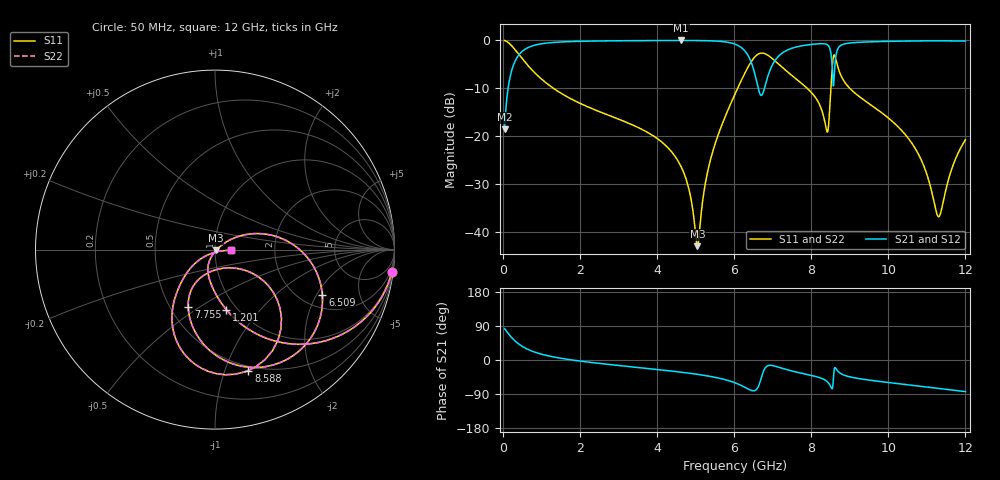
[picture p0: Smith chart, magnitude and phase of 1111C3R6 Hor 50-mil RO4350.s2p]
# GHz S MA R 50
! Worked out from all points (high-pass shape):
!   11951 points, 50 MHz to 12 GHz, reference 50 ohm
!   highest |S21| = -0.05 dB at 4.63 GHz (marker M1); lowest = -18.6 dB at 50 MHz (marker M2)
!   |S21| within 3 dB of the highest: 420.4 MHz to 6.354 GHz (5.933 GHz wide, 175 % of centre); 8.647 GHz to end of sweep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
!   lowest |S11| = -42.9 dB at 5.051 GHz (marker M3), VSWR 1.01, Z = 50.5 - j0.485 ohm
!   |S11| at or under -10 dB: 1.313 GHz to 6.094 GHz (4.782 GHz wide, 129 % of centre); 7.895 GHz to 8.512 GHz (617.2 MHz wide, 7.52 % of centre); 8.999 GHz to end of sweep
!   |S22| runs from -42.9 to -0.1 dB; largest |S21 - S12| = 0
!   S11 on the Smith chart (normalised r, x): 50 MHz: 1, -16; 1.201 GHz: 0.89, -0.68; 6.509 GHz: 2.57, -2.24; 7.755 GHz: 0.61, -0.45; 8.588 GHz: 0.46, -1.21; 12 GHz: 1.20, -0.01
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0.05  0.993 -7.1  0.1176 82.9  0.1176 82.9  0.993 -7.1
0.362  0.7599 -43.3  0.6496 46.6  0.6496 46.6  0.7599 -43.3
1.201  0.3407 -79.3  0.9391 10.6  0.9391 10.6  0.3407 -79.3
2.042  0.2167 -93.0  0.9748 -3.3  0.9748 -3.3  0.2167 -93.0
4.034  0.09293 -113.7  0.9928 -25.4  0.9928 -25.4  0.09293 -113.7
4.63  0.04785 -117.0  0.9943 -32.2  0.9943 -32.2  0.04785 -117.0
5.051  0.007152 -42.1  0.9926 -37.9  0.9926 -37.9  0.007152 -42.1
5.39  0.05705 34.3  0.986 -43.4  0.986 -43.4  0.05705 34.3
6.025  0.2749 18.8  0.9099 -60.2  0.9099 -60.2  0.2749 18.8
6.509  0.649 -22.9  0.4927 -81.2  0.4927 -81.2  0.649 -22.9
6.699  0.7334 -48.7  0.2663 -49.6  0.2663 -49.6  0.7334 -48.7
6.879  0.6966 -70.5  0.4237 -15.0  0.4237 -15.0  0.6966 -70.5
7.755  0.354 -114.9  0.8744 -35.1  0.8744 -35.1  0.354 -114.9
8.017  0.2821 -119.7  0.9054 -41.0  0.9054 -41.0  0.2821 -119.7
8.412  0.111 -83.8  0.8997 -56.5  0.8997 -56.5  0.111 -83.8
8.526  0.3944 -35.8  0.6604 -74.3  0.6604 -74.3  0.3944 -35.8
8.588  0.6992 -74.6  0.3642 -32.5  0.3642 -32.5  0.6992 -74.6
8.737  0.4648 -121.0  0.8641 -33.6  0.8641 -33.6  0.4648 -121.0
10.009  0.1539 -144.1  0.9734 -59.5  0.9734 -59.5  0.1539 -144.1
10.79  0.06404 -145.9  0.9833 -68.8  0.9833 -68.8  0.06404 -145.9
11.301  0.01449 -77.7  0.9851 -74.9  0.9851 -74.9  0.01449 -77.7
12  0.09167 -2.8  0.9806 -83.4  0.9806 -83.4  0.09167 -2.8
